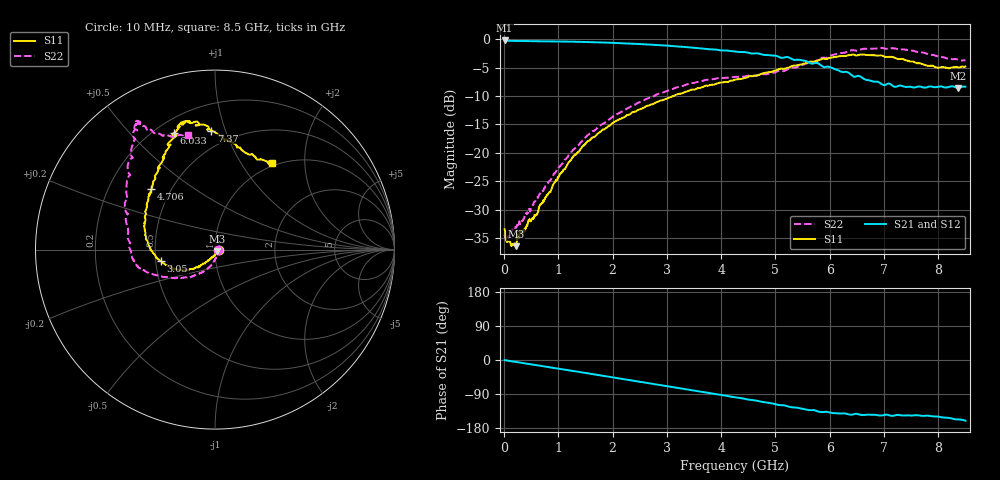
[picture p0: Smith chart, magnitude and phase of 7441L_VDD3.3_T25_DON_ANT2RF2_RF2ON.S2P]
!Agilent Technologies,E5071C,MY46417908,A.11.23
!Date: Mon May 03 19:54:00 2021
!Data & Calibration Information:
!Freq	S11:SOLT2(ON)	S21:SOLT2(ON)	S12:SOLT2(ON)	S22:SOLT2(ON)
!PortZ  Port1:50+j0  Port2:50+j0
!Above PortZ is port z conversion or system Z0 setting when saving the data.
!When reading, reference impedance value at option line is always used.
# Hz S dB R 50
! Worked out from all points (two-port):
!   1601 points, 10 MHz to 8.5 GHz, reference 50 ohm
!   highest |S21| = -0.21 dB at 10 MHz (marker M1); lowest = -8.6 dB at 8.362 GHz (marker M2)
!   |S21| within 3 dB of the highest: start of sweep to 5.088 GHz; 5.156 GHz to 5.248 GHz (91.85 MHz wide, 1.77 % of centre)
!   lowest |S11| = -36.5 dB at 216.9 MHz (marker M3), VSWR 1.03, Z = 51.2 - j0.922 ohm
!   |S11| at or under -10 dB: start of sweep to 3.119 GHz
!   |S22| runs from -35.2 to -1.5 dB; largest |S21 - S12| = 0.0057
!   S11 on the Smith chart (normalised r, x): 10 MHz: 1.04, -0.00; 3.05 GHz: 0.53, -0.08; 4.706 GHz: 0.39, +0.35; 6.033 GHz: 0.27, +0.67; 7.37 GHz: 0.38, +0.90; 8.5 GHz: 0.96, +1.37
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1e7  -33.50 -0.5  -0.21 -0.4  -0.21 -0.4  -34.69 -10.4
9.49e7  -35.62 -24.5  -0.27 -2.3  -0.27 -2.3  -34.69 -26.9
2.169438e8  -36.46 -36.8  -0.30 -5.2  -0.30 -5.1  -33.23 -41.8
5.83075e8  -31.03 -88.9  -0.34 -13.3  -0.34 -13.3  -28.47 -78.2
1.0288e9  -23.80 -117.8  -0.37 -23.4  -0.37 -23.4  -22.42 -99.7
1.426769e9  -19.10 -131.3  -0.46 -32.5  -0.46 -32.5  -18.06 -114.3
2.036988e9  -14.55 -142.6  -0.64 -46.6  -0.65 -46.6  -13.48 -133.7
2.843538e9  -10.97 -161.7  -1.03 -65.6  -1.04 -65.5  -9.62 -152.9
3.050481e9  -10.25 -167.8  -1.16 -70.4  -1.17 -70.4  -8.93 -156.5
3.708456e9  -8.21 171.4  -1.69 -85.9  -1.69 -85.9  -7.18 -166.8
4.255e9  -7.11 151.5  -2.16 -98.4  -2.17 -98.5  -6.62 -176.2
4.706031e9  -6.22 136.5  -2.55 -109.3  -2.51 -109.4  -6.22 172.9
5.257881e9  -4.94 122.1  -3.25 -123.7  -3.23 -123.4  -5.12 155.1
5.671769e9  -3.95 112.9  -4.30 -132.2  -4.26 -132.1  -4.01 139.1
6.032594e9  -3.25 109.3  -5.00 -139.6  -5.00 -139.3  -2.84 130.4
6.425256e9  -2.70 102.5  -6.48 -143.9  -6.48 -143.9  -1.91 123.8
6.541994e9  -2.72 105.2  -6.47 -143.8  -6.45 -143.6  -1.88 123.8
7.088538e9  -3.08 98.8  -7.79 -145.5  -7.81 -145.1  -1.66 121.8
7.369769e9  -3.56 91.7  -8.35 -146.6  -8.38 -146.1  -1.79 120.9
7.704062e9  -4.33 81.4  -8.43 -147.5  -8.45 -147.5  -2.31 119.3
8.362038e9  -4.93 58.6  -8.57 -156.8  -8.51 -156.5  -3.58 106.1
8.5e9  -4.80 56.8  -8.35 -160.3  -8.30 -159.8  -3.68 103.1
